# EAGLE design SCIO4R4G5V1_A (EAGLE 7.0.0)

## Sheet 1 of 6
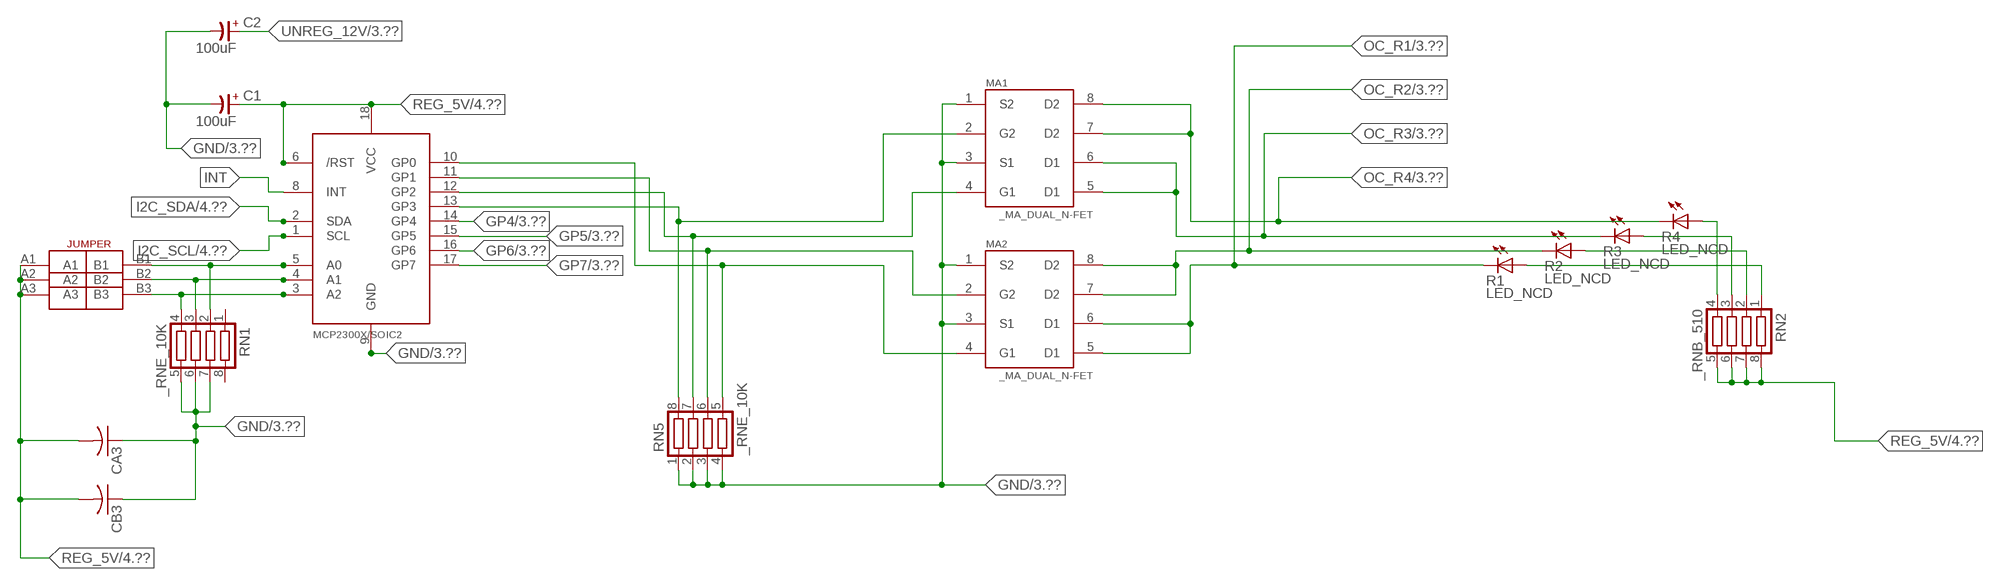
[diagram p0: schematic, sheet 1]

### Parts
C1  100uF  CP-E-025X060  [E-025X060]
C2  100uF  CP-E-025X060  [E-025X060]
CA3  CC1206KRX7R9BB104C1206K  [CC1206KRX7R9BB104]
CB3  TMK316F106ZL-TC1206K  [TMK316F106ZL-T]
IC2  MCP2300X/SO  [SO18W]
MA1  _MA_DUAL_N-FET  [_MA_DUAL_N-FET]
MA2  _MA_DUAL_N-FET  [_MA_DUAL_N-FET]
R1  LED_NCD  [CHIPLED_0603]
R2  LED_NCD  [CHIPLED_0603]
R3  LED_NCD  [CHIPLED_0603]
R4  LED_NCD  [CHIPLED_0603]
RN1  _RNE_10K  [RNE]
RN2  _RNB_510  [RNB]
RN5  _RNE_10K  [RNE]
U$18  JUMPER_3X2  [JUMPER_3X2]

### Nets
GND: C1.- C2.- CA3.1 CB3.1 IC2.9(GND) MA1.1(S2) MA1.3(S1) MA2.1(S2) MA2.3(S1) RN1.5 RN1.6 RN1.7 RN5.1 RN5.2 RN5.3 RN5.4 ; also sheet 3,4,6
GP4: IC2.14(GP4) ; also sheet 3
GP5: IC2.15(GP5) ; also sheet 3
GP6: IC2.16(GP6) ; also sheet 3
GP7: IC2.17(GP7) ; also sheet 3
I2C_SCL: IC2.1(SCL) ; also sheet 4
I2C_SDA: IC2.2(SDA) ; also sheet 4
INT: IC2.8(INT)
N$6: IC2.5(A0) RN1.2 U$18.B1
N$7: IC2.4(A1) RN1.3 U$18.B2
N$8: IC2.3(A2) RN1.4 U$18.B3
N$20: IC2.13(GP3) MA1.2(G2) RN5.8
N$21: IC2.12(GP2) MA1.4(G1) RN5.7
N$22: IC2.11(GP1) MA2.2(G2) RN5.6
N$23: IC2.10(GP0) MA2.4(G1) RN5.5
N$29: R4.A RN2.4
N$30: R3.A RN2.3
N$31: R2.A RN2.2
N$32: R1.A RN2.1
OC_R1: MA2.5(D1) MA2.6(D1) R1.C ; also sheet 3
OC_R2: MA2.7(D2) MA2.8(D2) R2.C ; also sheet 3
OC_R3: MA1.5(D1) MA1.6(D1) R3.C ; also sheet 3
OC_R4: MA1.7(D2) MA1.8(D2) R4.C ; also sheet 3
REG_5V: C1.+ CA3.2 CB3.2 IC2.6(/RST) IC2.18(VCC) RN2.5 RN2.6 RN2.7 RN2.8 U$18.A1 U$18.A2 U$18.A3 ; also sheet 4,6
UNREG_12V: C2.+ ; also sheet 3,4
Unconnected: RN1.1 RN1.8

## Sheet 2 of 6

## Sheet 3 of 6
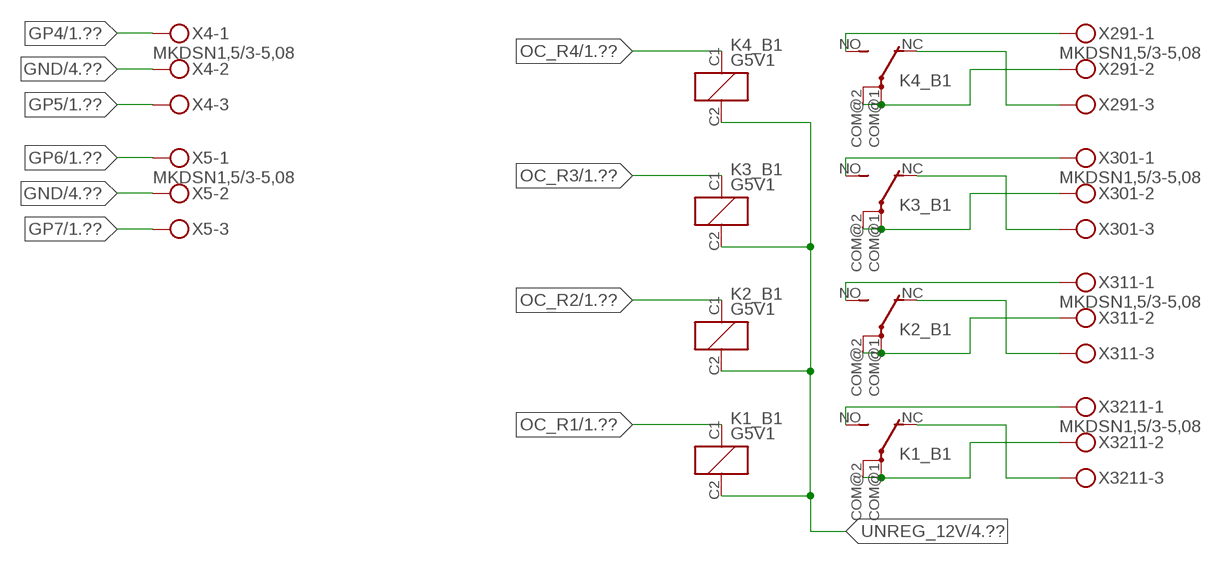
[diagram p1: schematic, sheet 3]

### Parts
K1_B1  G5V1  [G5V1]
K2_B1  G5V1  [G5V1]
K3_B1  G5V1  [G5V1]
K4_B1  G5V1  [G5V1]
X4  MKDSN1,5/3-5,08  [MKDSN1,5/3-5,08]
X5  MKDSN1,5/3-5,08  [MKDSN1,5/3-5,08]
X291  MKDSN1,5/3-5,08  [MKDSN1,5/3-5,08]
X301  MKDSN1,5/3-5,08  [MKDSN1,5/3-5,08]
X311  MKDSN1,5/3-5,08  [MKDSN1,5/3-5,08]
X3211  MKDSN1,5/3-5,08  [MKDSN1,5/3-5,08]

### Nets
GND: X4.2 X5.2 ; also sheet 1,4,6
GP4: X4.1 ; also sheet 1
GP5: X4.3 ; also sheet 1
GP6: X5.1 ; also sheet 1
GP7: X5.3 ; also sheet 1
N$215: K4_B1.NO(2:S) X291.1
N$216: K4_B1.NC(2:O) X291.3
N$217: K4_B1.COM@1(2:P) K4_B1.COM@2(2:P) X291.2
N$218: K3_B1.NO(2:S) X301.1
N$219: K3_B1.NC(2:O) X301.3
N$220: K3_B1.COM@1(2:P) K3_B1.COM@2(2:P) X301.2
N$221: K2_B1.NO(2:S) X311.1
N$222: K2_B1.NC(2:O) X311.3
N$223: K2_B1.COM@1(2:P) K2_B1.COM@2(2:P) X311.2
N$224: K1_B1.NO(2:S) X3211.1
N$225: K1_B1.NC(2:O) X3211.3
N$226: K1_B1.COM@1(2:P) K1_B1.COM@2(2:P) X3211.2
OC_R1: K1_B1.C1(1:C1) ; also sheet 1
OC_R2: K2_B1.C1(1:C1) ; also sheet 1
OC_R3: K3_B1.C1(1:C1) ; also sheet 1
OC_R4: K4_B1.C1(1:C1) ; also sheet 1
UNREG_12V: K1_B1.C2(1:C2) K2_B1.C2(1:C2) K3_B1.C2(1:C2) K4_B1.C2(1:C2) ; also sheet 1,4

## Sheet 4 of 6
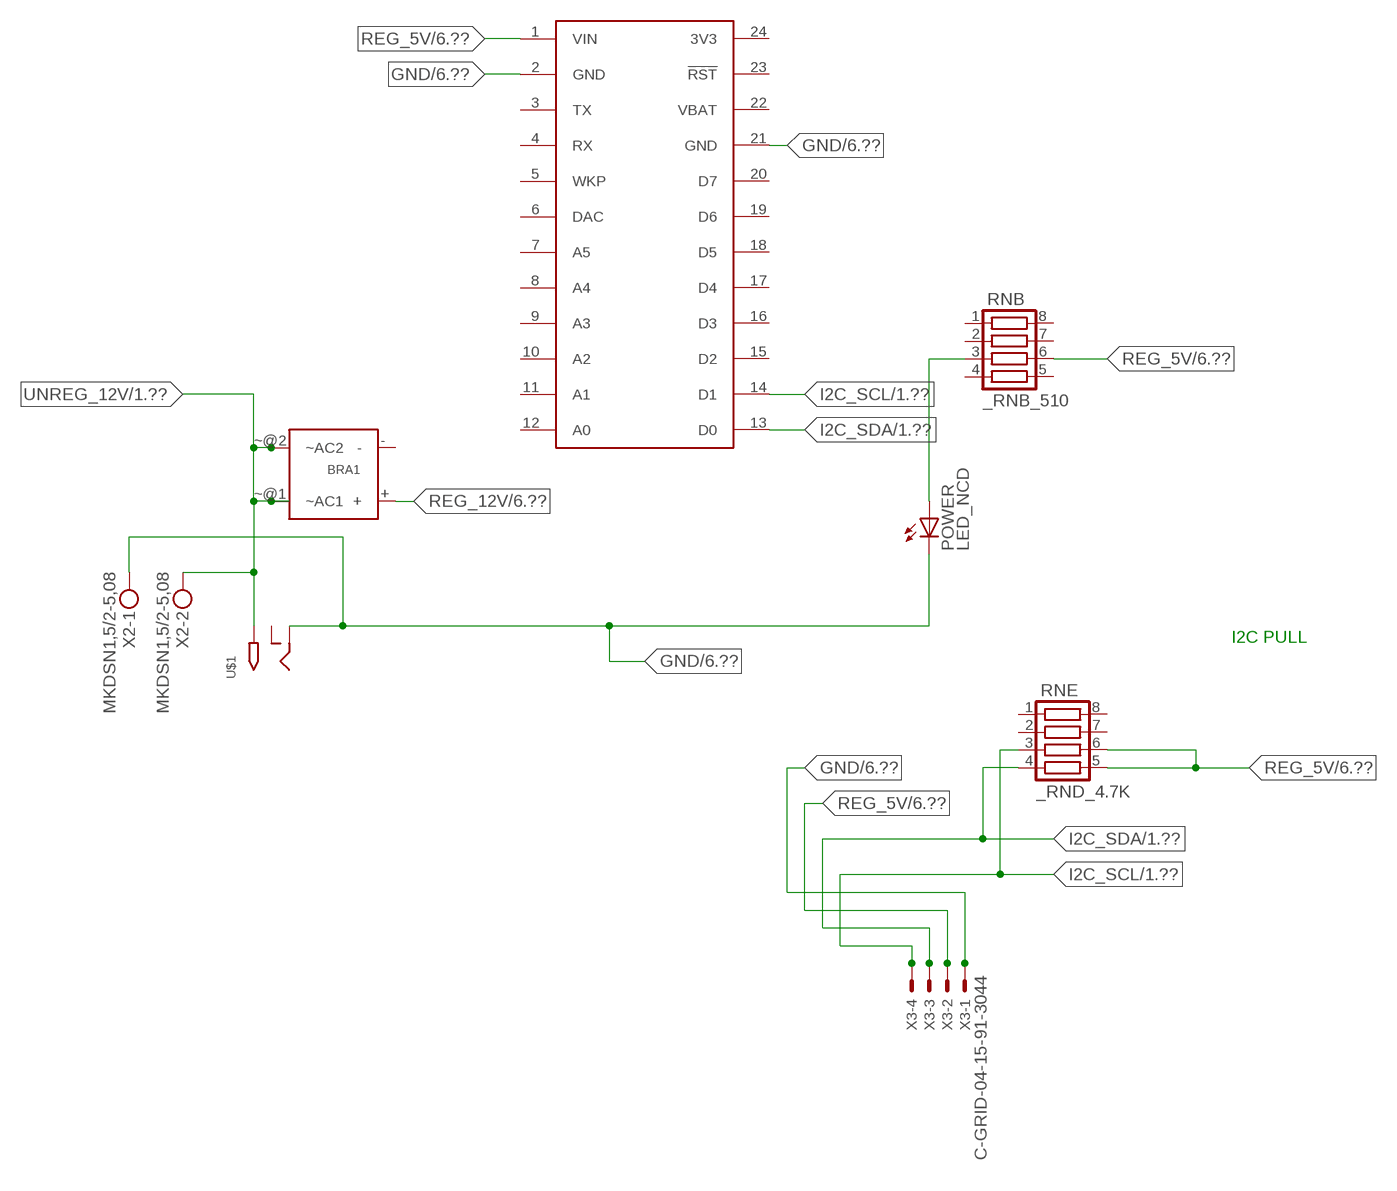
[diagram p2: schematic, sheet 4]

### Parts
BRA1  MB2S_  [MB2S]
POWER  LED_NCD  [CHIPLED_0603]
RNB  _RNB_510  [RNB]
RNE  _RND_4.7K  [RND]
S1  SPARK_CORECORE  [SPARK_CORE]
U$1  2.1MMJACK  [PJ-102A]
X2  MKDSN1,5/2-5,08  [MKDSN1,5/2-5,08]
X3  C-GRID-04-15-91-3044  [15-91-04]

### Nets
GND: POWER.C S1.2(GND) S1.21(GND) U$1.RING X2.1 X3.1 ; also sheet 1,3,6
I2C_SCL: RNE.3 S1.14(D1) X3.4 ; also sheet 1
I2C_SDA: RNE.4 S1.13(D0) X3.3 ; also sheet 1
N$2: POWER.A RNB.3
REG_5V: RNB.6 RNE.5 RNE.6 S1.1(VIN) X3.2 ; also sheet 1,6
REG_12V: BRA1.+ ; also sheet 6
UNREG_12V: BRA1.~@1(~AC1) BRA1.~@2(~AC2) U$1.TIP X2.2 ; also sheet 1,3
Unconnected: BRA1.- RNB.1 RNB.2 RNB.4 RNB.5 RNB.7 RNB.8 RNE.1 RNE.2 RNE.7 RNE.8 S1.3(TX) S1.4(RX) S1.5(WKP) S1.6(DAC) S1.7(A5) S1.8(A4) S1.9(A3) S1.10(A2) S1.11(A1) S1.12(A0) S1.15(D2) S1.16(D3) S1.17(D4) S1.18(D5) S1.19(D6) S1.20(D7) S1.23(!RST) U$1.RING_SW

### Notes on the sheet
- I2C PULL

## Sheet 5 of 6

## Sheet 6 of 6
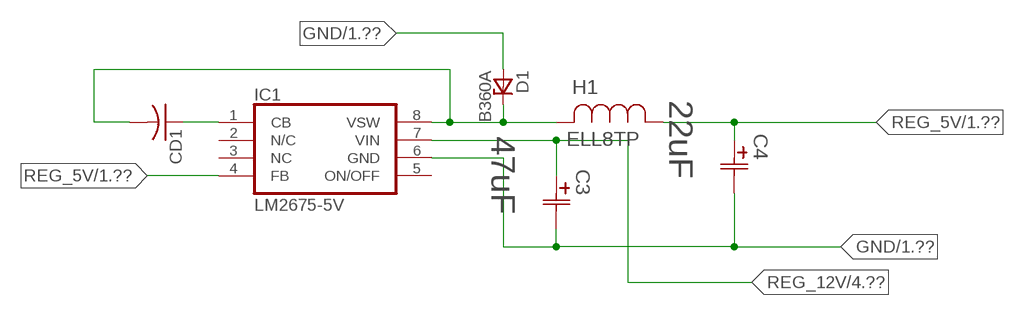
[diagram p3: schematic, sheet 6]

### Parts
C3  47uF  490-5463-6-NDCAP  [C2917(7343)-Y]
C4  22uF  490-5463-6-NDCAP  [C2917(7343)-Y]
CD1  _CD_10NF_50VC1206K  [_CD_10NF_50V]
D1  B360A  [DO214AC_ZENER]
H1  ELL8TP  [IND_ELL8TP]
IC1  LM2675-5V  LM2675  [SO-8]

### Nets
GND: C3.2(C2) C4.2(C2) D1.A IC1.6(GND) ; also sheet 1,3,4
N$1: CD1.2 D1.C H1.2 IC1.8(VSW)
N$3: CD1.1 IC1.1(CB)
REG_5V: C4.1(C1) H1.1 IC1.4(FB) ; also sheet 1,4
REG_12V: C3.1(C1) IC1.7(VIN) ; also sheet 4
Unconnected: IC1.2(N/C) IC1.5(ON/OFF)

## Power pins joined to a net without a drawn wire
3V3: S1.24(3V3)
NC: IC1.3(NC)
VBAT: S1.22(VBAT)

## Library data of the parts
BRA1 = NCD_ULTIMATE_LIBRARY:MB2S: Bridge Rectifier BRA MB2S 200V 500ma Digikey MB2S-TPMSTR-ND/MB2S-TP
C1 C2 = NCD_ULTIMATE_LIBRARY:CP-: Capacitors All Kinds POLARIZED CAP
C3 C4 = NCD_ULTIMATE_bhaskar:490-5463-6-ND: NCD CAP
CA3 = NCD_ULTIMATE_LIBRARY:CC1206KRX7R9BB104: Capacitor CA .1uF 50V SMT C1206K CC1206KRX7R9BB104
CB3 = NCD_ULTIMATE_LIBRARY:TMK316F106ZL-T: Capacitor CB 10uF SMT 1206 TMK316F106ZL-T
CD1 = NCD_ULTIMATE_LIBRARY:_CD_10NF_50V: Capacitor 10nF SMT
D1 = NCD_ULTIMATE_bhaskar:B360A: NCD DIODE B350A/B360A
H1 = NCD_ULTIMATE_bhaskar:ELL8TP: NCD coil
IC1 = NCD_ULTIMATE_bhaskar:LM2675: LM2675 NCD http://www.ti.com/lit/ds/symlink/lm2675.pdf
IC2 = NCD_ULTIMATE_LIBRARY:MCP2300X: Semiconductor Port Expander I/O 8-Bit I2C MCP23008 Inexpensive i2c i/o expander - 8 general purpose i/o pins with optional pullups
K1_B1 K2_B1 K3_B1 K4_B1 = NCD_ULTIMATE_LIBRARY:G5V1: RELAY 1 x switch, 0.5 A/125 V AC, 1 A/24 V DC , Omron
MA1 MA2 = NCD_ULTIMATE_LIBRARY:_MA_DUAL_N-FET: FET Dual N-Channel 8-SOIC NMOSFET Digikey 785-1064-2-ND/AO4842
POWER = NCD_ULTIMATE_bhaskar:LED_NCD
R1-R4 = NCD_ULTIMATE_LIBRARY:LED_NCD: LED Digikey 754-1132-2-ND/APT2012SRCPRV
RN1 RN5 = NCD_ULTIMATE_LIBRARY:_RNE_10K: Resistor Array RNE SMT 10K x 4 Single Resistor Source: http://www.ctscorp.com/components/Datasheets/CTSChipArrayDs.pdf Digikey 742C083103JPTR-ND/742C083103JP; OC_FARNELL: unknown; OC_NEWARK: unknown
RN2 RNB = NCD_ULTIMATE_LIBRARY:_RNB_510: Resistor Array RNB SMT 510 x 4 Single Resistor Source: http://www.ctscorp.com/components/Datasheets/CTSChipArrayDs.pdf Digikey 742C083511JPTR-ND/ 742C083511JP; OC_FARNELL: unknown; OC_NEWARK: unknown
RNE = NCD_ULTIMATE_LIBRARY:_RND_4.7K: Resistor Array RND SMT 4.7K x 4 Single Resistor Source: http://www.ctscorp.com/components/Datasheets/CTSChipArrayDs.pdf Digikey 742C083472JPTR-ND/742C083472JP; OC_FARNELL: unknown; OC_NEWARK: unknown
S1 = Spark:SPARK_CORE
U$1 = NCD_ULTIMATE_CONNECTORS:2.1MMJACK: 2.1mm x 5.5mm DC jack with internal switch. Digikey part #PJ-102A, 4UCON part #05537 By microbuilder.eu
U$18 = NCD_ULTIMATE_CONNECTORS:JUMPER_3X2
X2 = NCD_ULTIMATE_CONNECTORS:MKDSN1,5/2-5,08: MKDSN 1,5/ 2-5,08 Printklemme
X3 = NCD_ULTIMATE_CONNECTORS:C-GRID-04: CONNECTOR 4-Pos I2C wire to board 2.54 mm (0.100") pitch header Digikey WM1342-ND/0015912045; OC_FARNELL: unknown; OC_NEWARK: unknown
X4 X5 X291 X301 X311 X3211 = NCD_ULTIMATE_CONNECTORS:MKDSN1,5/3-5,08: MKDSN 1,5/ 3-5,08 Printklemme Nennstrom: 13,5 A Nennspannung: 250 V Rastermaß: 5,08 mm Polzahl: 3 Anschlussart: Schraubanschluss Montage: Löten Anschlussrichtung Leiter/Platine: 0 ° Artikelnummer: 1729131 Source: http://eshop.phoenixcontact.com .. 1729131.pdf

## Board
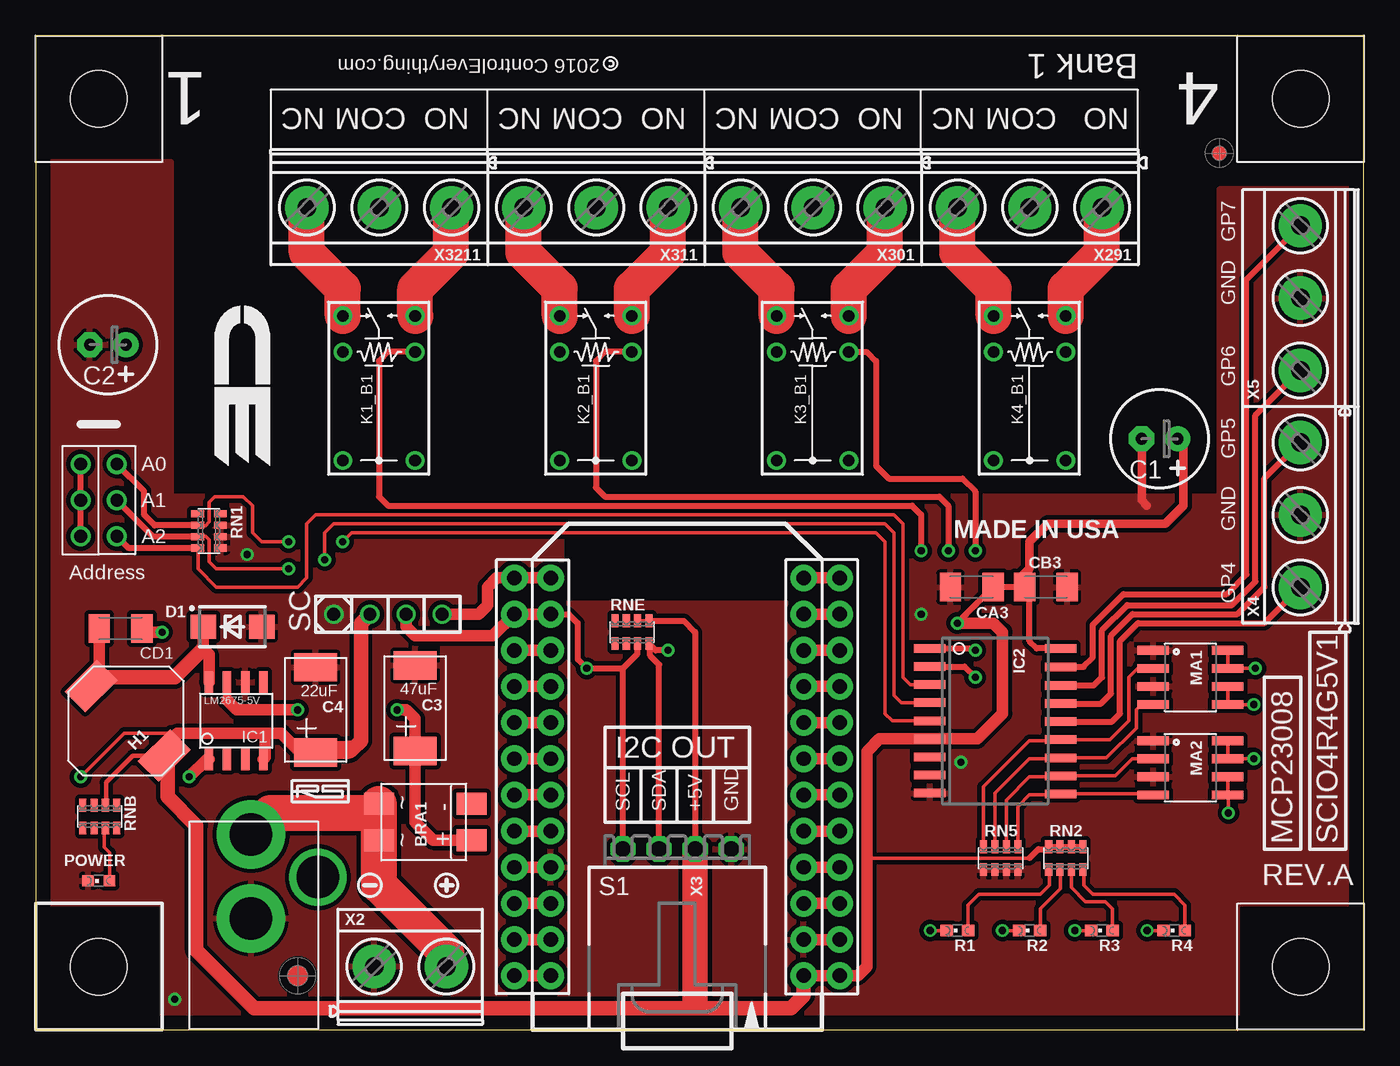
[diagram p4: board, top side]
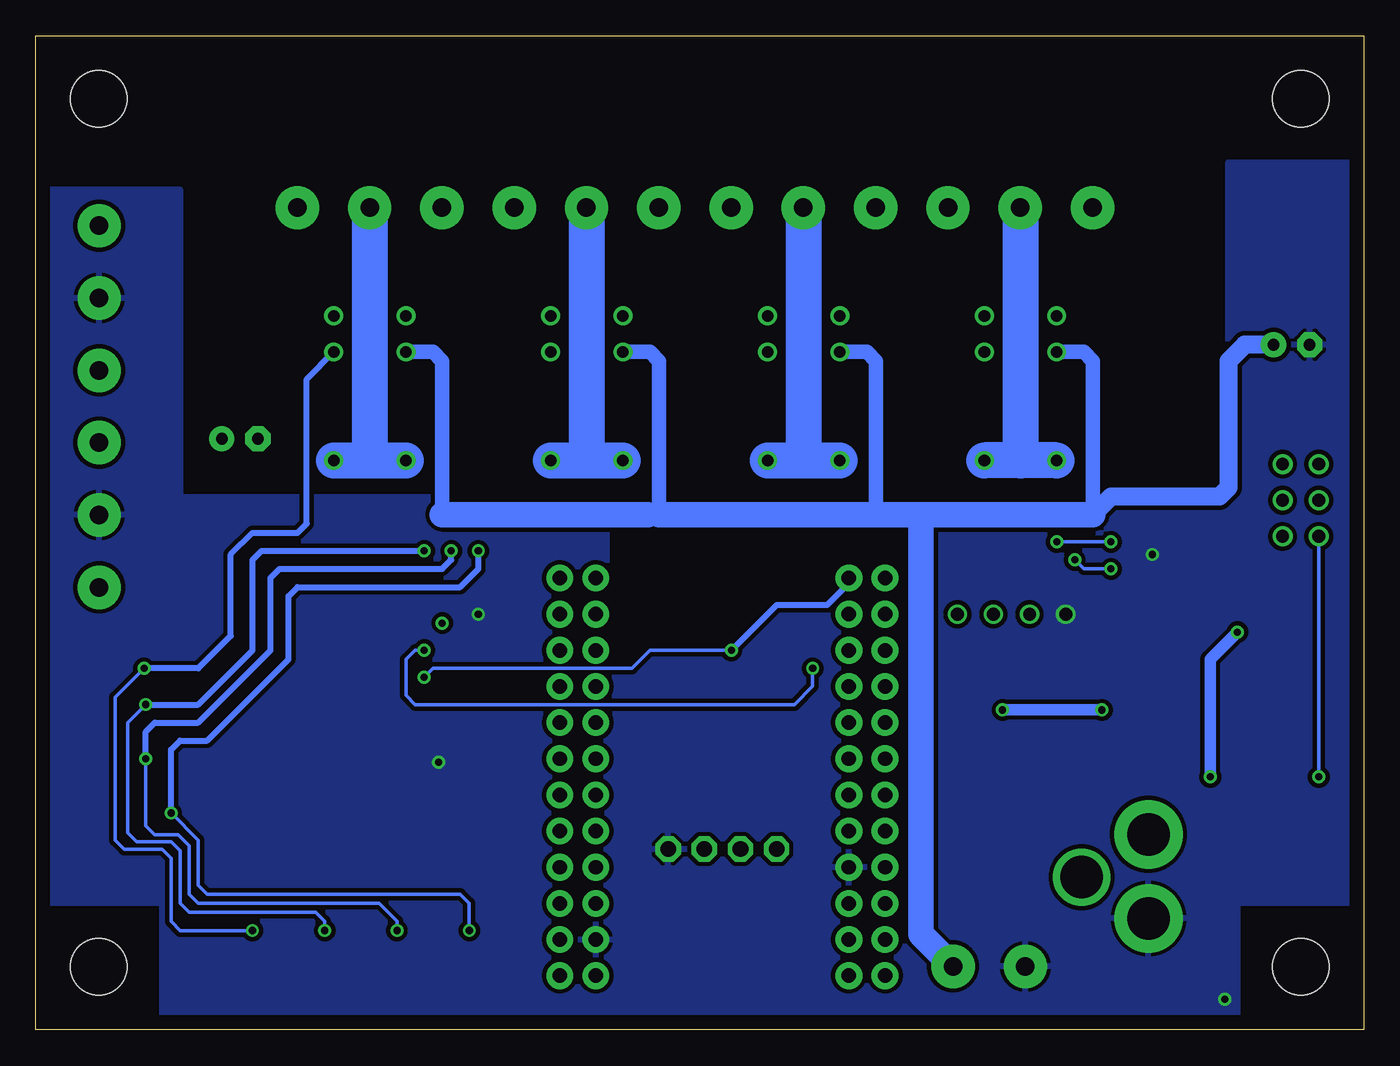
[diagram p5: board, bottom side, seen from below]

Size 93.34 x 69.85 mm. Coordinates in mm from the lower left corner, seen from the top.
Outline: 0,50.47 0,49.53
Outline: 0,49.53 0,0 78.74,0 93.34,0 93.34,69.85 0,69.85 0,49.53
Copper layers (1*16): Top 0.035mm / dielectric 1.5mm / Bottom 0.035mm
Design rules "default": minimum track width 10mil, minimum drill 24mil, track to track 8mil, track to pad 8mil, pad to pad 8mil, via to via 8mil, smd to smd 8mil, copper to edge 40mil, drill to drill 8mil, minimum pad ring 10mil, minimum via ring 8mil, stop-mask expansion 4mil, vias tented up to drill 0mil, thermal gap 10mil
Holes 3.96 mm at 4.45,4.45

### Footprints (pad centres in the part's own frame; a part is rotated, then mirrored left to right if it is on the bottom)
MB2S = smd 1.55 x 2.1: + 0,-6.5; - 2.54,-6.5; ~@1 0,0; ~@2 2.54,0
E-025X060 = drill 0.813 pad 1.778: + -1.27,0 | drill 0.813 pad 1.778 octagon: - 1.27,0
C2917(7343)-Y = smd 2 x 3: 1 -3,0; 2 3,0
CC1206KRX7R9BB104 = smd 1.5 x 2: 1 -1.5,0; 2 1.5,0
TMK316F106ZL-T = smd 1.5 x 2: 1 -1.5,0; 2 1.5,0
_CD_10NF_50V = smd 1.5 x 2: 1 -1.5,0; 2 1.5,0
DO214AC_ZENER = smd 1.8 x 1.7: A 2.05,0; C -2.05,0
IND_ELL8TP = smd 2.054 x 3.2 rotated 45: 1 -2.442,-2.696; 2 2.442,2.442
SO-8 = smd 0.6 x 1.55: 1 -1.905,-2.69; 2 -0.635,-2.69; 3 0.635,-2.69; 4 1.905,-2.69; 5 1.905,2.71; 6 0.635,2.71; 7 -0.635,2.71; 8 -1.905,2.71
SO18W = smd 0.6 x 2.2: 1 -4.445,-4.6; 2 -3.175,-4.6; 3 -1.905,-4.6; 4 -0.635,-4.6; 5 0.635,-4.6; 6 1.905,-4.6; 7 3.175,-4.6; 8 4.445,-4.6; 9 5.715,-4.6; 10 5.775,4.6; 11 4.505,4.6; 12 3.235,4.6; 13 1.965,4.6; 14 0.695,4.6; 15 -0.575,4.6; 16 -1.845,4.6; 17 -3.145,4.6; 18 -4.445,4.6
G5V1 = drill 0.813: C1 -2.54,2.54; C2 -2.54,-2.54; COM@1 5.08,-2.54; COM@2 5.08,2.54; NC -5.08,-2.54; NO -5.08,2.54
_MA_DUAL_N-FET = smd 0.61 x 2.21: 1 -1.905,-2.616; 2 -0.635,-2.616; 3 0.635,-2.616; 4 1.905,-2.616; 5 1.905,2.616; 6 0.635,2.616; 7 -0.635,2.616; 8 -1.905,2.616
CHIPLED_0603 = smd 0.8 x 0.8: A 0,-0.75; C 0,0.75
CHIPLED_0603' = smd 0.8 x 0.876: A 0,-0.75; C 0,0.75
RNE = smd 0.5 x 0.9: 1 -1.2,-0.8; 2 -0.4,-0.8; 3 0.4,-0.8; 4 1.2,-0.8; 5 1.2,0.8; 6 0.4,0.8; 7 -0.4,0.8; 8 -1.2,0.8
RNB = smd 0.5 x 0.9: 1 -1.2,-0.8; 2 -0.4,-0.8; 3 0.4,-0.8; 4 1.2,-0.8; 5 1.2,0.8; 6 0.4,0.8; 7 -0.4,0.8; 8 -1.2,0.8
RND = smd 0.5 x 0.9: 1 -1.2,-0.8; 2 -0.4,-0.8; 3 0.4,-0.8; 4 1.2,-0.8; 5 1.2,0.8; 6 0.4,0.8; 7 -0.4,0.8; 8 -1.2,0.8
SPARK_CORE = drill 1.016 pad 1.88: 1 -8.89,13.97; 2 -8.89,11.43; 3 -8.89,8.89; 4 -8.89,6.35; 5 -8.89,3.81; 6 -8.89,1.27; 7 -8.89,-1.27; 8 -8.89,-3.81; 9 -8.89,-6.35; 10 -8.89,-8.89; 11 -8.89,-11.43; 12 -8.89,-13.97; 13 8.89,-13.97; 14 8.89,-11.43; 15 8.89,-8.89; 16 8.89,-6.35; 17 8.89,-3.81; 18 8.89,-1.27; 19 8.89,1.27; 20 8.89,3.81; 21 8.89,6.35; 22 8.89,8.89; 23 8.89,11.43; 24 8.89,13.97; 25 -11.43,13.97; 26 -11.43,11.43; 27 -11.43,8.89; 28 -11.43,6.35; 29 -11.43,3.81; 30 -11.43,1.27; 31 -11.43,-1.27; 32 -11.43,-3.81; 33 -11.43,-6.35; 34 -11.43,-8.89; 35 -11.43,-11.43; 36 -11.43,-13.97; 37 11.43,13.97; 38 11.43,11.43; 39 11.43,8.89; 40 11.43,6.35; 41 11.43,3.81; 42 11.43,1.27; 43 11.43,-1.27; 44 11.43,-3.81; 45 11.43,-6.35; 46 11.43,-8.89; 47 11.43,-11.43; 48 11.43,-13.97
PJ-102A = drill 3 pad 4.8: RING 0.1,-3.39; TIP 0.1,-9.29 | drill 3 pad 3.251: RING_SW -4.6,-6.29
PCB_MOUNTING_HOLE = hole 3.962: 4.445,4.445
JUMPER_3X2 = drill 0.9: A1 0,5.08; A2 0,2.54; A3 0,0; B1 2.54,5.08; B2 2.54,2.54; B3 2.54,0
MKDSN1,5/2-5,08 = drill 1.3 pad 3.048: 1 -2.561,0.025; 2 2.519,0.025
15-91-04 = drill 1.1 pad 1.778 octagon: 1 -3.81,-7.62; 2 -1.27,-7.62; 3 1.27,-7.62; 4 3.81,-7.62
MKDSN1,5/3-5,08 = drill 1.3 pad 3.048: 1 -7.641,0.025; 2 -2.561,0.025; 3 2.519,0.025

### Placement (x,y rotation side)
BRA1  24.13,13.34 90 top
C1  78.99,41.53 180 top
C2  5.08,48.13 180 top
C3  26.67,22.61 90 top
C4  19.68,22.48 90 top
CA3  65.79,31.12 0 top
CB3  70.99,31.12 180 top
CD1  5.97,28.19 180 top
D1  13.84,28.32 0 top
H1  6.35,21.72 90 top
IC1  14.1,21.72 0 top
IC2  67.44,22.35 270 top
K1_B1  24.13,45.08 270 top
K2_B1  39.37,45.08 270 top
K3_B1  54.61,45.08 270 top
K4_B1  69.85,45.08 270 top
MA1  81.15,24.77 270 top
MA2  81.15,18.41 270 top
POWER  4.45,10.48 90 top
R1  LED_NCD  [CHIPLED_0603']  64.77,6.98 90 top
R2  LED_NCD  [CHIPLED_0603']  69.85,6.98 90 top
R3  LED_NCD  [CHIPLED_0603']  74.93,6.98 90 top
R4  LED_NCD  [CHIPLED_0603']  80.01,6.98 90 top
RN1  12.19,35.05 270 top
RN2  72.39,12.07 0 top
RN5  67.82,12.07 0 top
RNB  4.51,14.99 0 top
RNE  41.91,27.94 0 top
S1  45.09,17.78 180 top
U$1  15.24,4.45 180 top
U$4  PCB_MOUNTING_HOLE  [PCB_MOUNTING_HOLE]  93.34,60.96 90 top
U$6  PCB_MOUNTING_HOLE  [PCB_MOUNTING_HOLE]  93.34,0 90 top
U$10  [VISION_REF15]  18.41,3.81 0 top
U$11  PCB_MOUNTING_HOLE  [PCB_MOUNTING_HOLE]  8.89,60.96 90 top
U$18  3.17,34.67 0 top
U$19  [VISION_REF10]  83.19,61.59 0 top
U$21  [ICON_USA]  64.52,34.54 0 top
U$22  [ICON_MINUS]  23.5,10.16 180 top
U$24  [ICON_PLUS]  28.89,10.16 90 top
X2  26.35,4.45 0 top
X3  45.09,5.08 180 top
X4  88.9,38.73 90 top
X5  88.9,53.97 90 top
X291  67.31,57.78 180 top
X301  52.07,57.78 180 top
X311  36.83,57.78 180 top
X3211  21.59,57.78 180 top

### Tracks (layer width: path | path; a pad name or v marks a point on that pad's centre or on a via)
GND  (via drill 0.5, 0.9)
  Top 0.61: C1.- 77.72,37.21 78.11,36.83
  other vias: 14.86,33.4 65.02,18.8 9.78,2.16 20.95,29.21 62.23,29.21
  pour Bottom (isolate 0.305): -1.91,8.89 8.89,8.89 8.89,0 84.45,0 84.45,8.89 92.71,8.89 92.71,59.05 83.19,59.05 83.19,37.46 9.53,37.46 9.53,60.96 -1.91,60.96
  pour Top (isolate 0.305): -3.81,8.89 8.89,8.89 8.89,0 84.45,0 84.45,8.89 92.71,8.89 92.71,59.05 83.19,59.05 83.19,37.46 9.53,37.46 9.53,60.96 -3.81,60.96
GP4
  Top 0.406: IC2.14 75.63,21.66 76.2,22.23 76.2,27.3 77.47,28.57 86.36,28.57 X4.1
GP5
  Top 0.406: IC2.15 74.87,22.93 75.56,23.62 75.56,27.69 77.09,29.21 84.45,29.21 86.36,31.12 86.36,38.74 X4.3
GP6
  Top 0.406: IC2.16 74.36,24.2 74.93,24.77 74.93,28.07 76.71,29.85 84.07,29.85 85.72,31.5 85.72,43.18 X5.1
GP7
  Top 0.406: IC2.17 73.63,25.5 74.3,26.16 74.3,28.45 76.45,30.61 83.69,30.61 85.09,32 85.09,52.71 X5.3
I2C_SCL  (via drill 0.5, 0.9)
  Top 0.406: IC2.1 65.91,26.8 v66.04,26.67 | X3.4 41.27,25.4 | 41.27,25.4 42.29,26.42 42.29,27.12 RNE.3 | S1.14 37.47,29.21 38.1,28.57 38.1,26.04 v38.73,25.4 41.27,25.4
  Top 0.813: v26.04,29.21 26.04,28.32 26.67,27.69 32.13,27.69 33.66,29.21
  Bottom 0.254: v38.73,25.4 38.73,24.13 40.01,22.86 66.67,22.86 67.31,23.5 67.31,26.04 66.67,26.67 v66.04,26.67
I2C_SDA  (via drill 0.5, 0.9)
  Top 0.406: IC2.2 65.28,25.53 v66.04,24.77 | X3.3 43.81,25.65 43.18,26.29 43.18,27.07 RNE.4 43.58,26.67 v44.45,26.67
  Top 0.813: v28.57,29.21 31.11,29.21 31.75,29.85 31.75,31.12 32.38,31.75 33.66,31.75
  Bottom 0.254: v44.45,26.67 50.16,26.67 51.44,25.4 65.41,25.4 v66.04,24.77
  Bottom 0.406: S1.13 36.2,31.37 37.72,29.85 41.27,29.85 v44.45,26.67
N$1
  Top 0.813: H1.2 3.88,24.77 | D1.C 11.79,26.78 12.19,26.38 IC1.8 | CD1.2 4.47,24.79 4.45,24.77
  Top 1.016: 3.88,24.77 4.45,24.77 9.78,24.77 11.79,26.78
N$2
  Top 0.254: POWER.A 5.2,12.46 4.83,12.83 4.83,14.1 RNB.3
  Top 0.406: 4.95,14.14 RNB.3
N$3  (via drill 0.5)
  Top 0.813: IC1.1 12.04,19.03 v10.79,17.78 | v8.89,27.94 7.72,27.94 CD1.1
  Bottom 0.813: v10.79,17.78 10.79,26.04 v8.89,27.94
N$6  (via drill 0.5)
  Top 0.254: IC2.5 60.2,21.72 59.69,22.23 59.69,34.29 59.05,34.92 22.23,34.92 v21.59,34.29 | v17.78,34.29 15.88,34.29 15.24,34.92 15.24,36.83 14.61,37.46 12.57,37.46 12.19,37.08 12.19,35.69 11.94,35.43 11.41,35.43 RN1.2
  Top 0.406: RN1.2 8.36,35.45 7.62,36.2 7.62,37.85 U$18.B1
  Bottom 0.254: v21.59,34.29 v17.78,34.29
N$7  (via drill 0.5)
  Top 0.254: IC2.4 60.83,22.99 60.33,23.5 60.33,34.92 59.69,35.56 20.95,35.56 20.32,34.92 v20.32,33.02 | v17.78,32.38 12.7,32.38 12.19,32.89 12.19,34.42 11.94,34.67 11.41,34.67 RN1.3
  Top 0.406: RN1.3 8.27,34.65 U$18.B2
  Bottom 0.254: v20.32,33.02 19.68,32.38 v17.78,32.38
N$8
  Top 0.254: IC2.3 61.47,24.26 60.96,24.77 60.96,35.56 60.33,36.2 19.68,36.2 19.05,35.56 19.05,31.75 18.41,31.12 12.7,31.12 11.43,32.38 11.43,33.81 RN1.4
  Top 0.406: RN1.4 6.53,33.85 U$18.B3
N$20
  Top 0.254: MA1.2 77.47,25.4 76.83,24.77 76.83,21.72 75.5,20.39 IC2.13 71.97,20.32 69.85,20.32 66.62,17.09 RN5.8
N$21
  Top 0.254: MA1.4 77.72,22.86 77.34,22.48 77.34,21.21 75.25,19.12 IC2.12 71.97,19.05 69.85,19.05 67.42,16.62 RN5.7
N$22
  Top 0.254: MA2.2 77.09,19.05 75.89,17.85 IC2.11 71.97,17.78 69.85,17.78 68.22,16.15 RN5.6
N$23
  Top 0.254: MA2.4 78.6,16.58 IC2.10 71.97,16.51 69.85,16.51 69.02,15.68 RN5.5
N$29
  Top 0.254: R4.A 80.76,8.77 80.01,9.52 74.3,9.52 73.66,10.16 73.66,11.2 RN2.4
N$30
  Top 0.254: R3.A 75.68,8.52 75.18,9.02 73.79,9.02 72.77,10.03 72.77,11.25 RN2.3
N$31
  Top 0.254: R2.A 70.6,8.5 72.01,9.91 72.01,11.25 RN2.2
N$32
  Top 0.254: R1.A 65.52,8.75 66.29,9.52 70.61,9.52 71.25,10.16 71.25,11.21 RN2.1
N$215
  Top 2.54: K4_B1.NO 72.39,52.07 74.93,54.61 74.93,57.74 X291.1
N$216
  Top 2.54: K4_B1.NC 67.31,52.07 64.77,54.61 64.77,57.74 X291.3
N$217
  Bottom 2.54: X291.2 69.87,40.03 | 69.87,40.03 69.85,40 K4_B1.COM@1 | K4_B1.COM@2 69.89,40 69.87,40.03
N$218
  Top 2.54: K3_B1.NO 57.15,52.07 59.69,54.61 59.69,57.74 X301.1
N$219
  Top 2.54: K3_B1.NC 52.07,52.07 49.53,54.61 49.53,57.74 X301.3
N$220
  Bottom 2.54: K3_B1.COM@2 54.61,40 | 54.61,40 K3_B1.COM@1 | X301.2 54.63,40.03 54.61,40
N$221
  Top 2.54: K2_B1.NO 41.91,52.07 44.45,54.61 44.45,57.74 X311.1
N$222
  Top 2.54: K2_B1.NC 36.83,52.07 34.29,54.61 34.29,57.74 X311.3
N$223
  Bottom 2.54: K2_B1.COM@2 39.37,40 | 39.37,40 K2_B1.COM@1 | X311.2 39.39,40.03 39.37,40
N$224
  Top 2.54: K1_B1.NO 26.67,52.07 29.21,54.61 29.21,57.74 X3211.1
N$225
  Top 2.54: K1_B1.NC 21.59,52.07 19.05,54.61 19.05,57.74 X3211.3
N$226
  Bottom 2.54: K1_B1.COM@1 24.13,40 | 24.13,40 K1_B1.COM@2 | X3211.2 24.15,40.03 24.13,40
OC_R1  (via drill 0.5)
  Top 0.254: R1.C v62.87,6.98 | v83.82,15.24 83.82,16.43 MA2.5 MA2.6
  Top 0.406: v62.23,33.66 62.23,36.2 61.59,36.83 24.77,36.83 24.13,37.46 24.13,46.99 24.77,47.62 K1_B1.C1
  Bottom 0.254: v62.87,6.98 62.87,8.89 63.5,9.52 81.28,9.52 81.92,10.16 81.92,13.34 v83.82,15.24
  Bottom 0.406: v83.82,15.24 83.82,19.69 83.19,20.32 81.28,20.32 75.56,26.04 75.56,30.48 74.93,31.12 63.5,31.12 62.23,32.38 v62.23,33.66
OC_R2  (via drill 0.5)
  Top 0.254: R2.C v67.94,6.98 | v85.6,19.05 MA2.7 MA2.8
  Top 0.406: v64.14,33.66 64.14,36.83 63.5,37.46 40.01,37.46 39.37,38.1 39.37,46.99 40.01,47.62 K2_B1.C1
  Bottom 0.254: v67.94,6.98 67.94,7.62 69.22,8.89 81.92,8.89 82.55,9.52 82.55,12.95 83.31,13.72 84.96,13.72 85.6,14.35 v85.6,19.05
  Bottom 0.406: v85.6,19.05 85.6,20.96 84.96,21.59 81.92,21.59 76.83,26.67 76.83,31.75 76.2,32.38 64.77,32.38 64.14,33.02 v64.14,33.66
OC_R3  (via drill 0.5)
  Top 0.254: R3.C v73.03,6.98 | v85.6,22.86 MA1.5 MA1.6
  Top 0.406: K3_B1.C1 58.42,47.62 59.05,46.99 59.05,39.63 59.95,38.73 65.14,38.73 66.04,37.84 v66.04,33.66
  Bottom 0.254: v73.03,6.98 73.03,7.62 73.66,8.25 82.55,8.25 83.19,8.89 83.19,12.57 83.82,13.21 86.23,13.21 86.87,13.84 86.87,21.59 v85.6,22.86
  Bottom 0.406: v85.6,22.86 81.92,22.86 78.11,26.67 78.11,33.02 77.47,33.66 v66.04,33.66
OC_R4  (via drill 0.5)
  Top 0.254: R4.C v78.11,6.98 | v85.72,25.4 MA1.7 MA1.8
  Bottom 0.254: v78.11,6.98 83.19,6.98 83.82,7.62 83.82,12.07 84.45,12.7 87.12,12.7 87.76,13.34 87.76,23.37 v85.72,25.4
  Bottom 0.406: v85.72,25.4 81.92,25.4 79.63,27.69 79.63,33.4 78.11,34.92 74.93,34.92 74.3,35.56 74.3,45.72 K4_B1.C1
REG_5V  (via drill 0.5, 0.9)
  Top 0.229: 58.42,12.07 69.85,12.07
  Top 0.254: RNE.6 RNE.5 | 9.96,20.83 6.22,20.83 v3.17,17.78
  Top 0.305: H1.1 6.83,19.28 4.95,17.4 4.95,15.83 RNB.6
  Top 0.406: U$18.A3 U$18.A2 U$18.A1 | IC2.18 70.36,26.8 69.85,27.3 69.85,30.76 CB3.2 CA3.2 65.38,29.19 v64.77,28.57 | 62.71,20.32 IC2.6 | 69.85,12.07 70.48,12.7 71.03,12.7 RN2.8 RN2.7 RN2.6 RN2.5 | RNE.5 45.55,28.74 46.35,27.94 X3.2
  Top 0.61: CB3.2 69.22,31.39 69.22,31.75 69.85,32.38 69.85,34.29 71.12,35.56 79.38,35.56 80.64,36.83 80.64,41.15 C1.+
  Top 0.813: 16.13,20.83 9.96,20.83 H1.1 | 16.13,20.83 17.27,20.83 18.41,19.69 20.75,19.69 C4.1 | IC1.4 16.13,19.15 16.13,20.83 | S1.1 57.78,3.81 58.42,4.45 58.42,12.07 58.42,19.56 59.31,20.45 IC2.6 66.17,20.45 67.94,22.23 67.94,27.94 67.31,28.57 v64.77,28.57
  Top 1.016: 46.35,2.16 46.35,1.52 | 46.35,1.52 15.37,1.52 11.3,5.59 11.3,14.35 9.27,16.38 9.27,18.41 H1.1 | 22.05,19.69 22.23,19.69 22.86,20.32 22.86,28.57 v23.5,29.21 | S1.1 53.98,2.41 53.09,1.52 46.35,1.52
  Top 1.27: 20.75,19.69 22.05,19.69
  Top 1.778: X3.2 46.35,2.16
  Bottom 0.254: v3.17,17.78 U$18.A3
REG_12V  (via drill 0.5)
  Top 0.61: IC1.7 13.46,23.16 | 14.1,22.48 14.15,22.48
  Top 0.813: v18.41,22.48 14.15,22.48 13.46,23.16 | v25.4,22.48 26.04,22.48 26.67,21.84 C3.1 26.67,14.61 27.94,13.34 BRA1.+
  Bottom 0.813: v18.41,22.48 v25.4,22.48
UNREG_12V
  Top 2.54: X2.2 28.87,5.42 24.13,10.16 BRA1.~@1 24.13,15.24 | 24.13,15.24 BRA1.~@2 | U$1.TIP 15.14,13.87 16.51,15.24 24.13,15.24
  Bottom 1.016: K4_B1.C2 65.41,47.62 64.77,46.99 64.77,36.2 | K3_B1.C2 50.16,47.62 49.53,46.99 49.53,36.32 | 49.53,36.32 50.29,36.2 | 49.53,36.32 49.66,36.32 49.53,36.2 | K2_B1.C2 34.92,47.62 34.29,46.99 34.29,36.2 | K1_B1.C2 19.68,47.62 19.05,46.99 19.05,36.2
  Bottom 1.27: C2.+ 8.38,48.13 9.53,46.99 9.53,38.1 10.16,37.46 17.78,37.46 19.05,36.2
  Bottom 1.778: 49.53,36.2 34.29,36.2 31.11,36.2 | 31.11,36.2 19.05,36.2 | 64.77,36.2 50.29,36.2 | 31.11,36.2 31.11,6.71 X2.2

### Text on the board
tNames: 2016 ControlEverything.com | Bank 1 | 1 | 4 | NC | COM | NO | NC | COM | NO | NC | COM | NO | NC | COM | NO | GP7 | GND | GP6 | GP5 | A0 | A1 | GND | A2 | Address | GP4 | SC | I2C OUT | SCL | SDA | +5V | GND | MCP23008 | SCIO4R4G5V1 | REV.A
